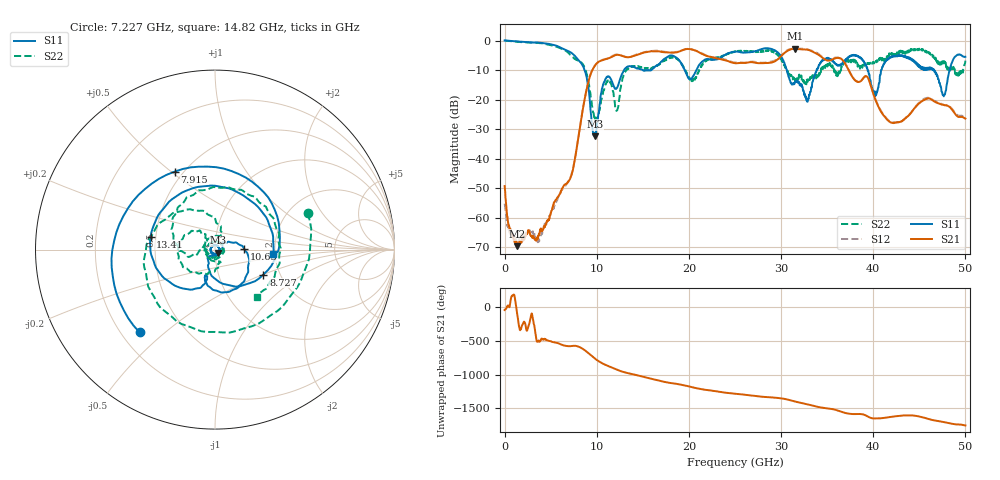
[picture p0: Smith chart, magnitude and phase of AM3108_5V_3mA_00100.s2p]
# Hz S DB R 50.0
!freq dBS11 angS11 dBS21 angS21 dBS12 angS12 dBS22 angS22
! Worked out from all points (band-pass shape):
!   1601 points, 10 MHz to 50 GHz, reference 50 ohm
!   highest |S21| = -2.78 dB at 31.53 GHz (marker M1); lowest = -69.6 dB at 1.385 GHz (marker M2)
!   |S21| within 3 dB of the highest: 11.46 GHz to 22.72 GHz (11.26 GHz wide, 65.9 % of centre); 29.84 GHz to 34.48 GHz (4.647 GHz wide, 14.4 % of centre)
!   lowest |S11| = -32.4 dB at 9.789 GHz (marker M3), VSWR 1.05, Z = 51.7 - j1.74 ohm
!   |S11| at or under -10 dB: 8.693 GHz to 12.97 GHz (4.274 GHz wide, 39.5 % of centre); 30.63 GHz to 33.85 GHz (3.221 GHz wide, 9.99 % of centre); 46.63 GHz to 48.29 GHz (1.66 GHz wide, 3.5 % of centre)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
!   |S22| runs from -27.5 to 0.0 dB; largest |S21 - S12| = 0.025
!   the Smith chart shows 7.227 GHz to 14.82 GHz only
!   S11 on the Smith chart (normalised r, x): 7.227 GHz: 0.27, -0.41; 7.915 GHz: 0.45, +0.51; 8.727 GHz: 1.64, -0.50; 10.63 GHz: 1.39, +0.01; 13.41 GHz: 0.47, +0.08; 14.82 GHz: 1.96, -0.11
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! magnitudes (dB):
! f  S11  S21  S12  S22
! 10 MHz  0.0  -49.3  -55.2  0.0
! 1.385 GHz  -0.3  -69.6  -68.9  -0.4
! 3.822 GHz  -0.7  -65.0  -67.3  -0.8
! 7.227 GHz  -4.1  -45.9  -45.6  -5.1
! 7.915 GHz  -6.2  -34.7  -34.5  -6.7
! 8.352 GHz  -7.8  -25.9  -25.9  -7.4
! 8.727 GHz  -10.4  -19.3  -19.2  -9.4
! 9.789 GHz  -32.4  -8.6  -8.5  -25.7
! 10.63 GHz  -15.7  -6.6  -6.5  -18.2
! 12.23 GHz  -15.9  -4.8  -4.7  -23.6
! 13.41 GHz  -8.7  -5.6  -5.6  -9.3
! 14.82 GHz  -9.7  -4.4  -4.2  -9.0
! 16.69 GHz  -8.1  -3.6  -3.4  -8.3
! 25 GHz  -3.8  -7.6  -7.4  -3.8
! 29.29 GHz  -3.2  -7.1  -6.8  -3.9
! 31.53 GHz  -14.1  -2.8  -2.7  -13.8
! 33.35 GHz  -15.6  -3.6  -3.4  -12.7
! 38 GHz  -4.8  -13.4  -13.4  -6.6
! 40.22 GHz  -18.8  -19.8  -19.7  -7.6
! 41.69 GHz  -6.0  -27.2  -27.1  -5.2
! 47.66 GHz  -18.9  -21.8  -21.8  -7.7
! 50 GHz  -5.5  -26.4  -26.5  -6.8
